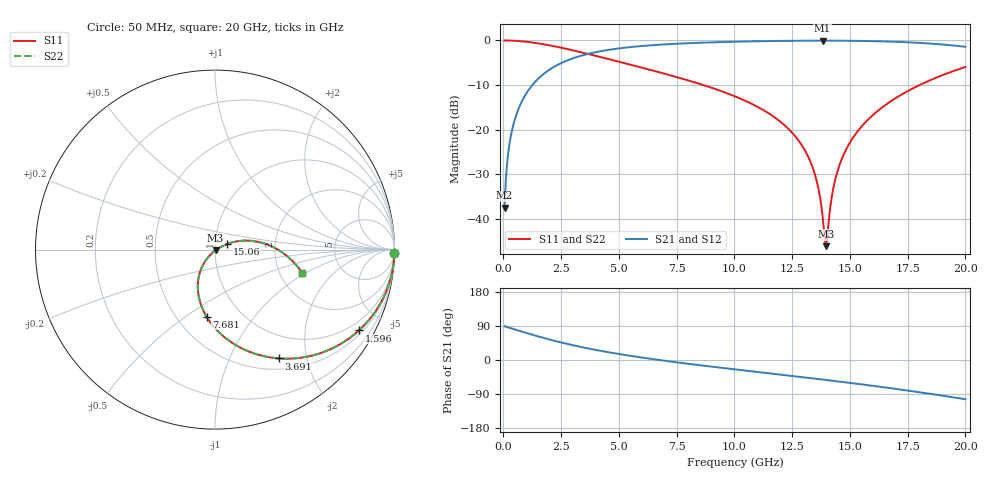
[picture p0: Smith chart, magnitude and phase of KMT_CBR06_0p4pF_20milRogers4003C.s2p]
! Data measured by Modelithics Inc. support@modelithics.com 813-866-6335
! KEMET CBR0603 0.4pF, Pad Width= 0.851mm, Pad Length= 0.64mm, Pad Gap= 0.62mm, 20mil Rogers 4003C substrate Data, January 2022
# hz S ma R 50
! 2 Port Network Data from SP1.SP block
! freq  magS11  angS11  magS21  angS21  magS12  angS12  magS22  angS22
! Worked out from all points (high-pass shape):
!   401 points, 50 MHz to 20 GHz, reference 50 ohm
!   highest |S21| = -0.05 dB at 13.82 GHz (marker M1); lowest = -37.5 dB at 50 MHz (marker M2)
!   |S21| within 3 dB of the highest: 3.636 GHz to end of sweep
!   lowest |S11| = -46.1 dB at 13.97 GHz (marker M3), VSWR 1.01, Z = 50.3 - j0.385 ohm
!   |S11| at or under -10 dB: 8.653 GHz to 18.02 GHz (9.365 GHz wide, 70.2 % of centre)
!   |S22| runs from -46.1 to 0.0 dB; largest |S21 - S12| = 0
!   S11 on the Smith chart (normalised r, x): 50 MHz: open; 1.596 GHz: 0.64, -3.72; 3.691 GHz: 0.65, -1.55; 7.681 GHz: 0.69, -0.60; 15.06 GHz: 1.15, +0.07; 20 GHz: 2.66, -0.94
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5e7  0.9999 -1.0  0.01328 89.0  0.01328 89.0  0.9999 -1.0
2.495e8  0.9978 -4.8  0.06613 85.2  0.06613 85.2  0.9978 -4.8
4.98875e8  0.9913 -9.5  0.1314 80.5  0.1314 80.5  0.9913 -9.5
9.4775e8  0.9695 -17.9  0.2445 72.1  0.2445 72.1  0.9695 -17.9
1.596125e9  0.9196 -29.3  0.3919 60.6  0.3919 60.6  0.9196 -29.3
3.391625e9  0.7338 -55.9  0.6777 34.0  0.6777 34.0  0.7338 -55.9
3.690875e9  0.7026 -59.6  0.7098 30.2  0.7098 30.2  0.7026 -59.6
5.13725e9  0.5653 -75.4  0.8226 14.4  0.8226 14.4  0.5653 -75.4
6.73325e9  0.4405 -89.6  0.895 0.0  0.895 0.0  0.4405 -89.6
7.680875e9  0.3766 -97.1  0.9234 -7.6  0.9234 -7.6  0.3766 -97.1
1.0025e10  0.236 -114.0  0.9681 -24.8  0.9681 -24.8  0.236 -114.0
1.22195e10  0.1091 -128.0  0.9895 -40.2  0.9895 -40.2  0.1091 -128.0
1.291775e10  0.06684 -131.4  0.993 -45.1  0.993 -45.1  0.06684 -131.4
1.336662e10  0.03888 -131.5  0.9942 -48.3  0.9942 -48.3  0.03888 -131.5
1.3616e10  0.02313 -128.3  0.9945 -50.1  0.9945 -50.1  0.02313 -128.3
1.38155e10  0.01083 -115.0  0.9946 -51.6  0.9946 -51.6  0.01083 -115.0
1.396512e10  0.004933 -50.8  0.9946 -52.7  0.9946 -52.7  0.004933 -50.8
1.426438e10  0.0208 20.9  0.9942 -54.9  0.9942 -54.9  0.0208 20.9
1.4414e10  0.03078 24.3  0.9938 -56.0  0.9938 -56.0  0.03078 24.3
1.506238e10  0.07604 24.9  0.9909 -60.9  0.9909 -60.9  0.07604 24.9
1.670825e10  0.2029 14.0  0.9714 -73.9  0.9714 -73.9  0.2029 14.0
2e10  0.5045 -15.2  0.8486 -103.6  0.8486 -103.6  0.5045 -15.2
